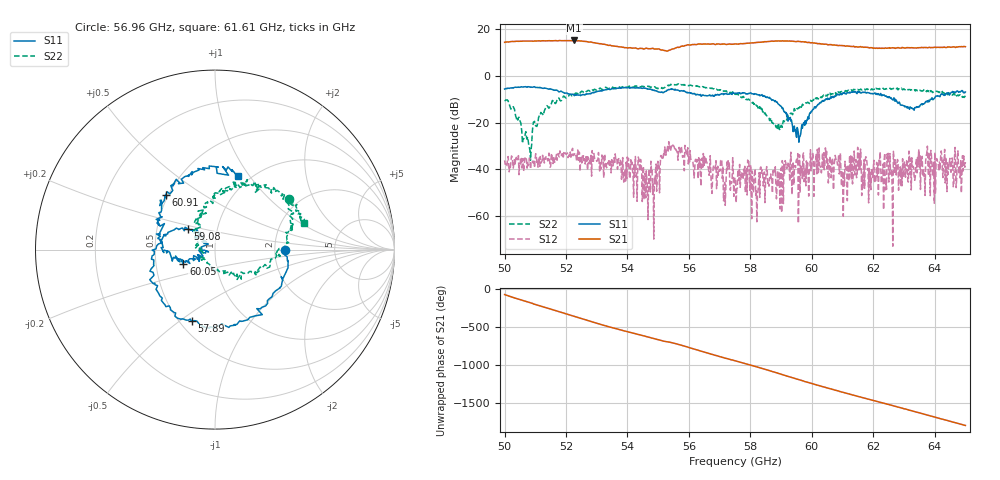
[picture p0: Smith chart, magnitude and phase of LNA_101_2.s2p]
! Created Tue Jul 15 12:32:12 2008
# hz S ma R 50
! 2 Port Network Data from blockName block
! freq  magS11  angS11  magS21  angS21  magS12  angS12  magS22  angS22
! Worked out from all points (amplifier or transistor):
!   801 points, 50 GHz to 65 GHz, reference 50 ohm
!   highest |S21| = 15.3 dB at 52.27 GHz (marker M1)
!   |S21| within 3 dB of that: 55.66 GHz to 61.82 GHz (6.161 GHz wide, 10.5 % of centre)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
!   unconditionally stable (mu >= 1): start of sweep to end of sweep
!   at 52.49 GHz: K = 3.47, MAG = 16.7 dB, |S12| = -35.0 dB
!   at 57.5 GHz: K = 10.89, MAG = 15.5 dB, |S12| = -43.8 dB
!   at 65 GHz: K = 5.74, MAG = 14.2 dB, |S12| = -36.9 dB
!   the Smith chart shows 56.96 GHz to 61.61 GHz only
!   S11 on the Smith chart (normalised r, x): 56.96 GHz: 2.29, -0.01; 57.89 GHz: 0.57, -0.56; 59.08 GHz: 0.72, +0.17; 60.05 GHz: 0.69, -0.11; 60.91 GHz: 0.48, +0.36; 61.61 GHz: 0.88, +0.89
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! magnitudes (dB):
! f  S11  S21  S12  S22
! 50 GHz  -5.6  14.5  -36.2  -10.3
! 50.81 GHz  -4.7  15.0  -35.2  -30.6
! 51.35 GHz  -5.3  15.1  -34.4  -13.2
! 52.27 GHz  -8.4  15.3  -33.8  -7.8
! 52.51 GHz  -8.1  15.0  -37.3  -6.5
! 54.41 GHz  -5.2  11.9  -40.9  -4.5
! 54.61 GHz  -5.4  12.0  -40.7  -4.6
! 55.01 GHz  -6.8  11.7  -39.5  -5.3
! 55.42 GHz  -5.5  11.4  -31.0  -3.7
! 56.96 GHz  -8.1  13.8  -42.6  -6.0
! 57.5 GHz  -7.3  13.8  -43.8  -7.8
! 57.89 GHz  -7.5  14.1  -51.1  -10.1
! 58.23 GHz  -7.9  14.4  -50.6  -12.9
! 59.08 GHz  -14.4  15.0  -54.7  -19.2
! 59.56 GHz  -24.5  14.9  -63.2  -13.6
! 60.01 GHz  -14.9  14.3  -35.5  -10.7
! 60.05 GHz  -14.3  14.3  -36.5  -10.3
! 60.91 GHz  -7.7  13.1  -39.5  -6.8
! 61.61 GHz  -7.3  12.5  -37.1  -5.7
! 62.51 GHz  -9.0  12.1  -45.5  -5.2
! 63.31 GHz  -14.1  12.1  -39.1  -6.0
! 65 GHz  -6.8  12.6  -36.9  -8.4
